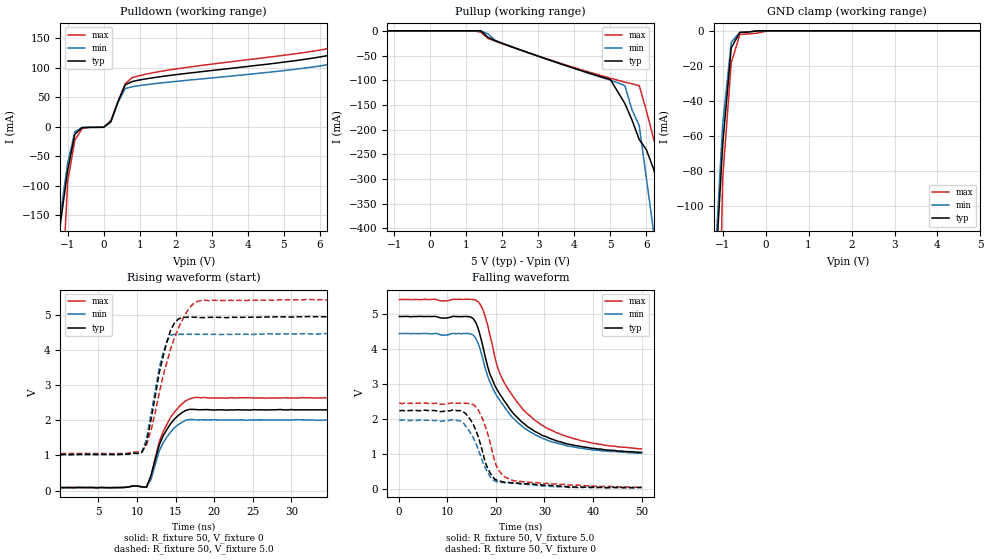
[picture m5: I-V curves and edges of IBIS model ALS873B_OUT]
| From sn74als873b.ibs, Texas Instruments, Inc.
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|   Model ALS873B_OUT
[Model]   ALS873B_OUT
Model_type  3-state
Polarity   Non-Inverting
Enable   Active-Low
Vref =   0
Rref =   500
Cref =   50p
Vmeas =   1.3
| variable   typ   min   max
C_comp   4.044pf   3.934pf   4.107pf
[Temperature Range]   25   0   70
[Voltage Range]   5.0   4.5   5.5
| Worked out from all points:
|   slope of the pulldown table from 0 to 0.75 V, typ, clamps not added: 9.84 ohm
|   GND clamp passes 1 mA (typ) near -0.60 V on its own axis
|   rising waveform, R_fixture 50, V_fixture 0: 20-80 % time 2.26ns typ, 2.2ns min, 2.46ns max; typ from 0.086 V to 2.29 V
|   falling waveform, R_fixture 50, V_fixture 5.0: 20-80 % time 9.02ns typ, 9ns min, 9.23ns max; typ from 4.93 V to 1.06 V
|   rising waveform, R_fixture 50, V_fixture 5.0: 20-80 % time 2.18ns typ, 1.79ns min, 3.21ns max; typ from 1.02 V to 4.95 V
|   falling waveform, R_fixture 50, V_fixture 0: 20-80 % time 3.23ns typ, 3.66ns min, 3.29ns max; typ from 2.24 V to 0.058 V
[Pulldown]
|   Voltage   I(typ)   I(min)   I(max)
-5V       -1.869A    -2.023A    -1.73A
-1.4V     -270.6mA   -250.8mA   -399.7mA
-1.2V     -163.3mA   -149mA     -332.9mA
-1V       -73.52mA   -61.28mA   -92.86mA
-800mV    -12.38mA   -8.287mA   -22.53mA
-600mV    -1.178mA   -788.9uA   -2.741mA
200mV     9.236mA    7.787mA    10.66mA
600mV     71.41mA    65.14mA    73.45mA
800mV     76.99mA    68.16mA    83.72mA
6.2V      120.6mA    105.2mA    132.3mA
8.4V      157.7mA    138.8mA    168.9mA
10V       186.8mA    165.4mA    197.7mA
[Pullup]
|   Voltage   I(typ)   I(min)   I(max)
-5V       688.3nA    720.4nA    827.5nA
1.4V      -87.11uA   -5.317uA   -3.03mA
2V        -25.56mA   -24.96mA   -26.24mA
5V        -98.67mA   -99.93mA   -95.92mA
5.4V      -147.1mA   -111.1mA   -103.8mA
5.8V      -220.1mA   -192mA     -111mA
6V        -240.9mA   -299.4mA   -162mA
6.2V      -280.1mA   -406.7mA   -219mA
6.6V      -385.4mA   -613.4mA   -310.3mA
6.8V      -465.9mA   -714.2mA   -371.8mA
7V        -559.5mA   -815mA     -440.6mA
10V       -1.94A     -2.328A    -1.568A
[GND Clamp]
|   Voltage   I(typ)   I(min)   I(max)
-5V       -1.964A    -2.116A    -1.763A
-1.2V     -151.5mA   -140.7mA   -319.7mA
-1V       -64.92mA   -53.61mA   -84.26mA
-800mV    -9.669mA   -6.534mA   -18.3mA
-600mV    -926.7uA   -731.8uA   -2.044mA
-200mV    -42.07uA   -20.13uA   -1.338mA
99.48fV   816.5nA    742.2nA    -200.9uA
200mV     841.7nA    749nA      438.3nA
5V        842.2nA    751.6nA    711.5nA
[Ramp]
| variable   typ   min   max
dV/dt_r  1.350E+00/2.291E-09  1.176E+00/2.270E-09  1.534E+00/2.451E-09
dV/dt_f  2.462E+00/7.873E-09  2.190E+00/8.134E-09  2.718E+00/7.708E-09
R_load = 50
[Rising Waveform]
R_fixture = 50
V_fixture = 0
V_fixture_min = 0
V_fixture_max = 0
C_fixture = 0pf
L_fixture = 0nH
|   Time   V(typ)   V(min)   V(max)
97.66ps   85.76mV    87.13mV    87.28mV
9.473ns   131.7mV    136.1mV    128.9mV
11.23ns   99.18mV    89.88mV    97.66mV
11.82ns   426.8mV    319.2mV    412.8mV
12.89ns   1.296V     1.125V     1.386V
13.38ns   1.552V     1.354V     1.671V
14.36ns   1.902V     1.662V     2.084V
15.82ns   2.215V     1.94V      2.46V
17.29ns   2.308V     2.019V     2.636V
50ns      2.289V     2.004V     2.625V
[Falling Waveform]
R_fixture = 50
V_fixture = 5.0
V_fixture_min = 4.5
V_fixture_max = 5.5
C_fixture = 0pf
L_fixture = 0nH
|   Time   V(typ)   V(min)   V(max)
97.66ps   4.934V     4.442V     5.416V
14.36ns   4.93V      4.448V     5.424V
15.82ns   4.77V      4.313V     5.4V
17.29ns   4.094V     3.727V     5.137V
18.75ns   3.292V     3.064V     4.41V
19.73ns   2.974V     2.777V     3.806V
21.68ns   2.532V     2.363V     3.052V
26.56ns   1.784V     1.684V     2.148V
35.84ns   1.267V     1.214V     1.455V
50ns      1.057V     1.035V     1.156V
[Rising Waveform]
R_fixture = 50
V_fixture = 5.0
V_fixture_min = 4.5
V_fixture_max = 5.5
C_fixture = 0pf
L_fixture = 0nH
|   Time   V(typ)   V(min)   V(max)
97.66ps   1.02V      1.025V     1.054V
10.64ns   1.084V     1.092V     1.111V
11.23ns   1.362V     1.463V     1.292V
11.82ns   2.011V     2.183V     1.708V
12.89ns   3.349V     3.484V     2.776V
13.87ns   4.216V     4.231V     3.636V
15.33ns   4.869V     4.441V     4.596V
16.8ns    4.93V      4.44V      5.193V
17.77ns   4.924V     4.44V      5.368V
50ns      4.953V     4.467V     5.438V
[Falling Waveform]
R_fixture = 50
V_fixture = 0
V_fixture_min = 0
V_fixture_max = 0
C_fixture = 0pf
L_fixture = 0nH
|   Time   V(typ)   V(min)   V(max)
97.66ps   2.244V     1.969V     2.463V
12.4ns    2.248V     1.964V     2.463V
13.87ns   2.147V     1.785V     2.456V
15.33ns   1.854V     1.472V     2.417V
17.29ns   1.047V     773.8mV    1.998V
18.26ns   612mV      498.4mV    1.603V
20.21ns   260.8mV    213.3mV    634.5mV
21.68ns   206.5mV    192.6mV    366.7mV
24.12ns   179.9mV    172.9mV    239.1mV
50ns      57.83mV    51.73mV    58.59mV
